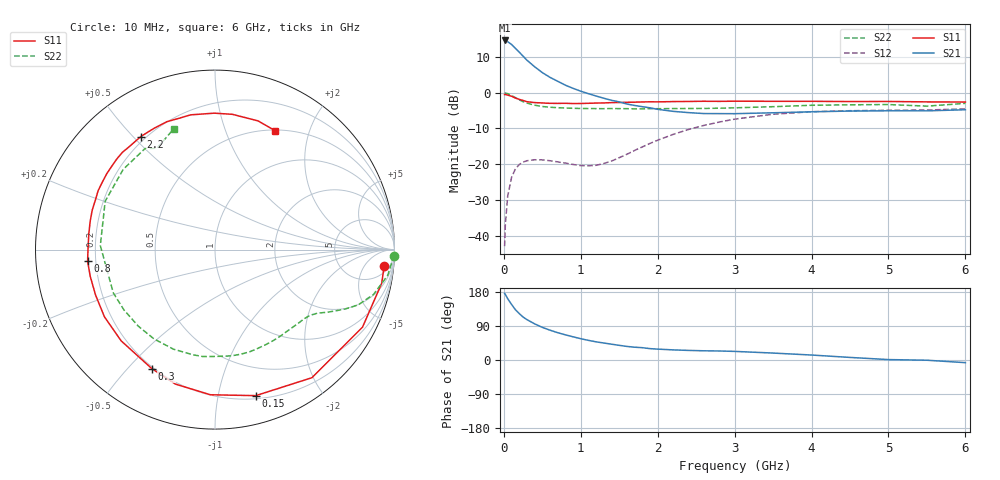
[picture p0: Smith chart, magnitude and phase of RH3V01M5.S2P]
! SIEMENS Small Signal Semiconductors
! BFR106
! Si NPN RF Bipolar Junction Transistor in SOT23
! VCE = 3 V  IC = 1.5 mA
! Common Emitter S-Parameters:  August  1996
# GHz  S  MA  R  50
!  f  S11  S21  S12  S22
! GHz  MAG  ANG  MAG  ANG  MAG  ANG  MAG  ANG
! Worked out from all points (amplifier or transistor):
!   36 points, 10 MHz to 6 GHz, reference 50 ohm
!   highest |S21| = 14.7 dB at 10 MHz (marker M1)
!   |S21| within 3 dB of that: start of sweep to 187.8 MHz
!   unconditionally stable (mu >= 1): 827.5 MHz to 2.082 GHz; 3.137 GHz to end of sweep
!   at 250 MHz: K = 0.29, MSG = 14.8 dB, |S12| = -19.4 dB
!   at 1.4 GHz: K = 1.35, MAG = 5.0 dB, |S12| = -19.1 dB
!   at 6 GHz: K = 1.02, MAG = -1.0 dB, |S12| = -4.5 dB
!   S11 on the Smith chart (normalised r, x): 10 MHz: 9, -16; 150 MHz: 0.23, -1.29; 300 MHz: 0.19, -0.59; 800 MHz: 0.17, -0.04; 2.2 GHz: 0.18, +0.53; 6 GHz: 0.51, +1.51
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0.01  0.9469 -5.6  5.414 175.8  0.0071 86.6  0.9994 -1.9
0.02  0.9476 -11.4  5.376 172.9  0.0146 85.7  0.9906 -3.5
0.05  0.9285 -27.7  5.193 161.7  0.0355 74.2  0.973 -8.5
0.1  0.8949 -52.9  4.766 146.8  0.0651 61.8  0.9178 -15.8
0.15  0.8448 -74.4  4.199 132.7  0.0858 50.0  0.8552 -21.1
0.2  0.8092 -91.8  3.721 122.6  0.0988 42.3  0.7995 -24.4
0.25  0.7811 -106.4  3.26 113.3  0.107 35.7  0.7506 -27.1
0.3  0.7509 -117.9  2.863 106.6  0.1118 31.5  0.7186 -29.0
0.4  0.7293 -135.8  2.32 95.4  0.1154 24.9  0.6708 -31.9
0.5  0.7209 -148.7  1.92 86.1  0.1149 21.5  0.6428 -34.8
0.6  0.712 -159.2  1.647 78.7  0.1118 19.7  0.6277 -38.1
0.8  0.7128 -174.8  1.279 66.4  0.1037 21.8  0.6114 -45.3
1.1  0.7131 167.2  0.972 51.8  0.0948 36.2  0.6019 -57.8
1.6  0.7365 145.0  0.696 35.8  0.1379 65.0  0.5992 -81.1
2.2  0.7535 123.3  0.55 26.7  0.2613 66.6  0.6011 -112.6
2.8  0.7585 105.2  0.511 23.8  0.3891 53.7  0.6085 -146.5
3.5  0.7602 90.3  0.525 18.3  0.5008 36.4  0.6393 178.0
4  0.7599 82.7  0.542 13.1  0.5435 24.7  0.6687 156.2
4.5  0.7544 76.7  0.555 6.8  0.5614 14.8  0.6792 138.8
5  0.7561 71.5  0.56 1.1  0.5695 6.8  0.6848 124.7
5.5  0.746 66.6  0.559 -0.6  0.5736 3.1  0.6507 119.8
6  0.7425 63.1  0.579 -7.0  0.5964 -4.7  0.7115 108.8
